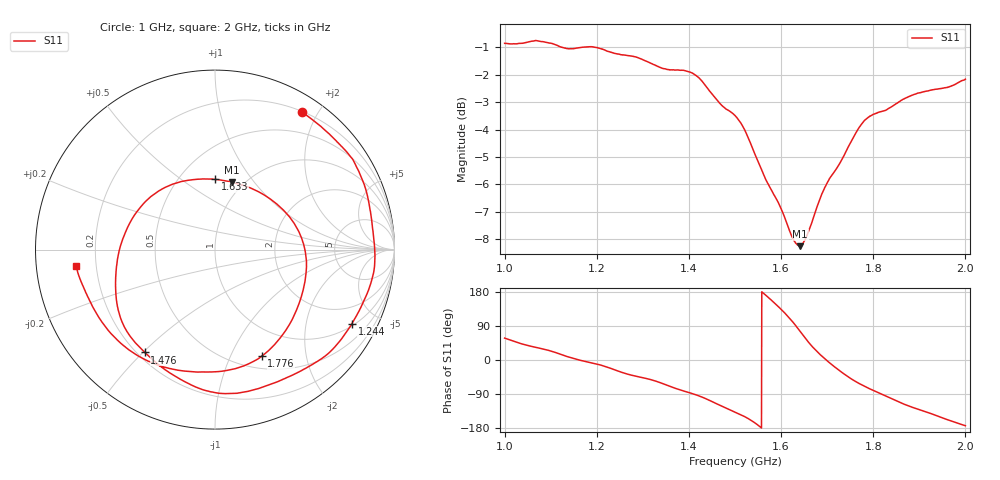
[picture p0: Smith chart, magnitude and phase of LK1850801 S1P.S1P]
!Agilent Technologies,E5071C,
!Date:
!Data & Calibration Information:
!Freq	S11:SOLT1(ON)
!PortZ  Port1:50+j0
!Above PortZ is port z conversion or system Z0 setting when saving the data.
!When reading, reference impedance value at option line is always used.
# Hz S dB R 50
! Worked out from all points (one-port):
!   1601 points, 1 GHz to 2 GHz, reference 50 ohm
!   lowest |S11| = -8.3 dB at 1.641 GHz (marker M1), VSWR 2.26, Z = 44.4 + j39.1 ohm
!   |S11| at or under -10 dB: nowhere
!   S11 on the Smith chart (normalised r, x): 1 GHz: 0.21, +1.79; 1.244 GHz: 1.10, -3.65; 1.476 GHz: 0.23, -0.51; 1.633 GHz: 0.74, +0.68; 1.776 GHz: 0.64, -1.32; 2 GHz: 0.12, -0.06
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1e9  -0.85 57.8
1.05625e9  -0.78 36.5
1.09375e9  -0.83 25.9
1.125e9  -1.00 13.6
1.191875e9  -0.98 -8.2
1.244375e9  -1.24 -28.4
1.25e9  -1.25 -30.8
1.278125e9  -1.32 -40.9
1.32e9  -1.60 -52.7
1.375e9  -1.82 -76.6
1.42375e9  -2.15 -95.6
1.475625e9  -3.18 -124.3
1.5e9  -3.49 -137.3
1.533125e9  -4.47 -157.9
1.564375e9  -5.72 173.5
1.5975e9  -6.79 136.8
1.625e9  -7.95 100.9
1.6325e9  -8.15 89.6
1.64125e9  -8.25 75.7
1.669375e9  -7.25 33.1
1.69375e9  -6.16 4.5
1.71875e9  -5.46 -20.6
1.75e9  -4.49 -48.0
1.77625e9  -3.76 -66.4
1.81875e9  -3.33 -90.6
1.875e9  -2.82 -120.4
1.9425e9  -2.51 -149.2
2e9  -2.16 -173.4
